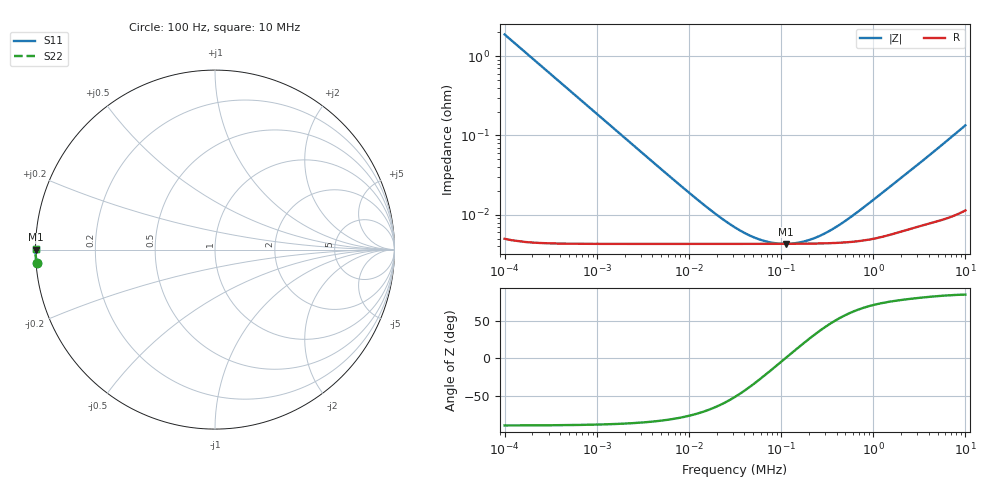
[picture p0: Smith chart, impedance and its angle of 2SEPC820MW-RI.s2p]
!  *** S-Parameter ***
!  Copyright (C) Panasonic Industry
!  Conductive Polymer Aluminum Solid Capacitors (OS-CON)
!  Parts No. 2SEPC820MW
! Touchstone file from project
# GHZ S RI R 50.000000
! Modal data exported
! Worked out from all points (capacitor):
!   401 points, 100 Hz to 10 MHz, reference 50 ohm
!   read as one part in shunt: C = 850 uF near 105.9 Hz
!   lowest |Z| = 4.31 mohm at 112.2 kHz (marker M1)
!   series resonance near 111.4 kHz, so ESL is about 2.4 nH
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1e-07  -0.9942 -0.0744  0.00577 -0.0744  0.00577 -0.0744  -0.9942 -0.0744
! Port Impedance 5.000000E+001 0.000000E+000 5.000000E+001 0.000000E+000
1.059254e-07  -0.9948 -0.0703  0.00517 -0.0703  0.00517 -0.0703  -0.9948 -0.0703
2.304093e-07  -0.9988 -0.0325  0.00123 -0.0325  0.00123 -0.0325  -0.9988 -0.0325
6.878599e-07  -0.9997 -0.0109  0.000291 -0.0109  0.000291 -0.0109  -0.9997 -0.0109
4.731513e-06  -0.9998 -0.00158  0.000175 -0.00158  0.000175 -0.00158  -0.9998 -0.00158
9.440609e-06  -0.9998 -0.000787  0.000173 -0.000787  0.000173 -0.000787  -0.9998 -0.000787
1.539927e-05  -0.9998 -0.000477  0.000172 -0.000477  0.000172 -0.000477  -0.9998 -0.000477
2.304093e-05  -0.9998 -0.000311  0.000172 -0.000311  0.000172 -0.000311  -0.9998 -0.000311
3.162278e-05  -0.9998 -0.000218  0.000172 -0.000218  0.000172 -0.000218  -0.9998 -0.000218
4.340103e-05  -0.9998 -0.000146  0.000172 -0.000146  0.000172 -0.000146  -0.9998 -0.000146
5.956621e-05  -0.9998 -8.98e-05  0.000172 -8.98e-05  0.000172 -8.98e-05  -0.9998 -8.98e-05
8.17523e-05  -0.9998 -4.23e-05  0.000172 -4.23e-05  0.000172 -4.23e-05  -0.9998 -4.23e-05
0.0001122018  -0.9998 9.19e-07  0.000172 9.19e-07  0.000172 9.19e-07  -0.9998 9.19e-07
0.0001539927  -0.9998 4.42e-05  0.000173 4.42e-05  0.000173 4.42e-05  -0.9998 4.42e-05
0.0002175204  -0.9998 9.66e-05  0.000174 9.66e-05  0.000174 9.66e-05  -0.9998 9.66e-05
0.0003072557  -0.9998 0.00016  0.000175 0.00016  0.000175 0.00016  -0.9998 0.00016
0.000459727  -0.9998 0.00026  0.000179 0.00026  0.000179 0.00026  -0.9998 0.00026
0.0007286182  -0.9998 0.000424  0.000188 0.000424  0.000188 0.000424  -0.9998 0.000424
0.001496236  -0.9998 0.000864  0.000224 0.000864  0.000224 0.000864  -0.9998 0.000864
0.003868121  -0.9997 0.00213  0.00031 0.00213  0.00031 0.00213  -0.9997 0.00213
0.009440609  -0.9995 0.00505  0.000465 0.00505  0.000465 0.00505  -0.9995 0.00505
0.01  -0.9995 0.00534  0.000483 0.00534  0.000483 0.00534  -0.9995 0.00534
